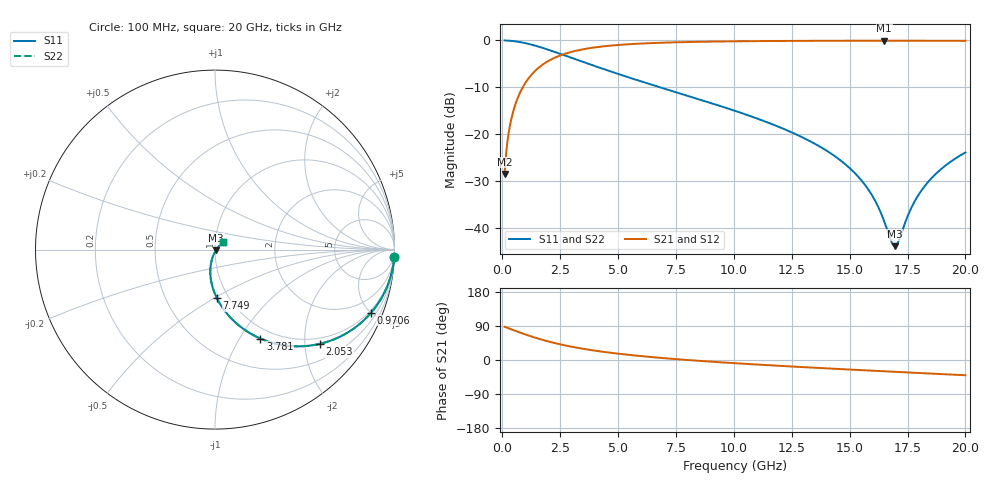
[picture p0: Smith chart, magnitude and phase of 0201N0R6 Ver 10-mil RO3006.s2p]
# GHz S MA R 50
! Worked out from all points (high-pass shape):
!   1601 points, 100 MHz to 20 GHz, reference 50 ohm
!   highest |S21| = -0.06 dB at 16.49 GHz (marker M1); lowest = -28.5 dB at 100 MHz (marker M2)
!   |S21| within 3 dB of the highest: 2.579 GHz to end of sweep
!   lowest |S11| = -43.8 dB at 16.95 GHz (marker M3), VSWR 1.01, Z = 50.5 - j0.343 ohm
!   |S11| at or under -10 dB: 6.822 GHz to end of sweep
!   |S22| runs from -43.8 to 0.0 dB; largest |S21 - S12| = 0
!   S11 on the Smith chart (normalised r, x): 100 MHz: 1, -49; 970.6 MHz: 0.85, -5.01; 2.053 GHz: 0.85, -2.34; 3.781 GHz: 0.86, -1.23; 7.749 GHz: 0.88, -0.51; 20 GHz: 1.09, +0.10
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0.1  0.9993 -2.3  0.03771 87.6  0.03771 87.6  0.9993 -2.3
0.274125  0.9947 -6.4  0.1029 83.6  0.1029 83.6  0.9947 -6.4
0.4358125  0.9867 -10.2  0.1623 79.8  0.1623 79.8  0.9867 -10.2
0.672125  0.9691 -15.5  0.2461 74.5  0.2461 74.5  0.9691 -15.5
0.970625  0.9384 -22.0  0.3446 68.0  0.3446 68.0  0.9384 -22.0
2.052688  0.786 -41.9  0.6162 48.0  0.6162 48.0  0.786 -41.9
3.420812  0.5978 -59.4  0.7987 30.3  0.7987 30.3  0.5978 -59.4
3.7815  0.5562 -63.0  0.8279 26.7  0.8279 26.7  0.5562 -63.0
6.741625  0.3208 -83.1  0.9428 6.1  0.9428 6.1  0.3208 -83.1
7.749062  0.2689 -87.9  0.9585 1.1  0.9585 1.1  0.2689 -87.9
10.05  0.1778 -96.9  0.9788 -8.5  0.9788 -8.5  0.1778 -96.9
13.37081  0.08249 -106.1  0.9905 -20.1  0.9905 -20.1  0.08249 -106.1
15.34838  0.0359 -106.5  0.9929 -26.3  0.9929 -26.3  0.0359 -106.5
15.99512  0.02183 -101.7  0.9931 -28.3  0.9931 -28.3  0.02183 -101.7
16.49263  0.01186 -87.5  0.9932 -29.8  0.9932 -29.8  0.01186 -87.5
16.69162  0.008558 -72.2  0.9932 -30.4  0.9932 -30.4  0.008558 -72.2
16.95281  0.006435 -31.8  0.9931 -31.2  0.9931 -31.2  0.006435 -31.8
17.1145  0.007305 -4.0  0.9931 -31.7  0.9931 -31.7  0.007305 -4.0
17.7115  0.01739 34.3  0.9929 -33.5  0.9929 -33.5  0.01739 34.3
18.209  0.02739 40.9  0.9925 -35.0  0.9925 -35.0  0.02739 40.9
19.005  0.04369 43.7  0.9918 -37.3  0.9918 -37.3  0.04369 43.7
20  0.0641 43.5  0.9905 -40.2  0.9905 -40.2  0.0641 43.5
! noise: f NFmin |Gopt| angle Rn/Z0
0.1  0.001113  0.9693  1.133  0.008219
2.301  0.005382  0.8284  5.486  0.006585
4.515  0.008295  0.7855  9.39  0.007897
6.729  0.01081  0.7586  13.34  0.008945
8.943  0.01311  0.7391  17.27  0.00984
11.14  0.01527  0.7243  21.16  0.01063
13.36  0.01734  0.7127  25.03  0.01136
15.57  0.01936  0.7035  28.85  0.01204
17.79  0.02134  0.6964  32.61  0.01268
20  0.0233  0.6908  36.32  0.01329
